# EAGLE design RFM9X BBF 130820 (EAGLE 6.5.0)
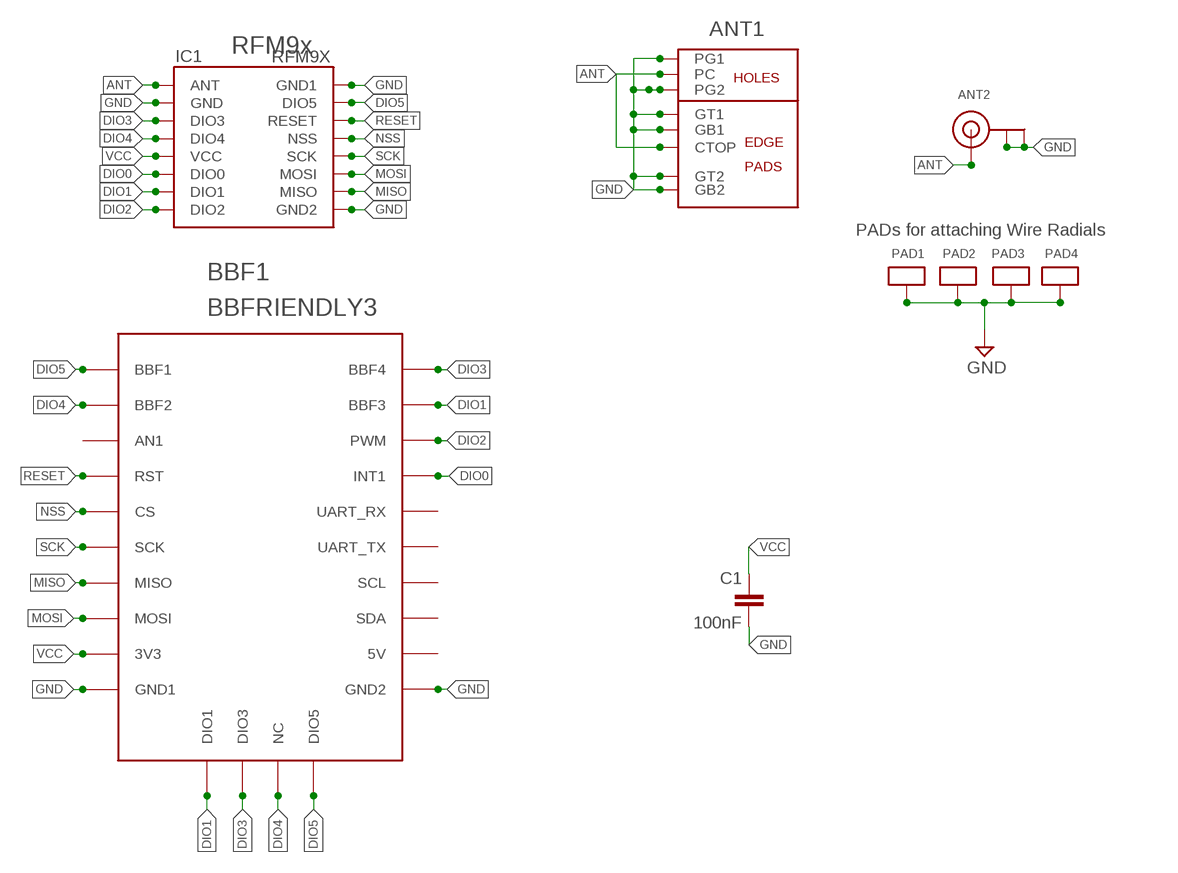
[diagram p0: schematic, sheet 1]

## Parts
ANT1  CUSTOMSMA  [CUSTOMSMA]
ANT2  ANTENNA_U.FL  [U.FL]
BBF1  BBFRIENDLY3  [PCB_SOCKET_BBFRIENDLY3]
C1  100nF  C-EUC1206  [C1206]
IC1  RFM9X  RFM98_PIH  [RFM98_PIH]
PAD1  ANTPAD2  [ANTPAD2]
PAD2  ANTPAD2  [ANTPAD2]
PAD3  ANTPAD2  [ANTPAD2]
PAD4  ANTPAD2  [ANTPAD2]

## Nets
ANT: ANT1.CTOP ANT1.PC ANT2.3(SIGNAL) IC1.ANT
DIO0: BBF1.INT(INT1) IC1.DIO0
DIO1: BBF1.BBF3 BBF1.DIO1 IC1.DIO1
DIO2: BBF1.PWM IC1.DIO2
DIO3: BBF1.BBF4 BBF1.DIO3 IC1.DIO3
DIO4: BBF1.BBF2 BBF1.NC IC1.DIO4
DIO5: BBF1.BBF1 BBF1.DIO5 IC1.DIO5
GND [VDD]: ANT1.G1 ANT1.G2 ANT1.GB1 ANT1.GB2 ANT1.GT1 ANT1.GT2 ANT2.1(GND) ANT2.2(GND) BBF1.GND1 BBF1.GND2 C1.2 IC1.GND IC1.GND1 IC1.GND2 PAD1.P$1 PAD2.P$1 PAD3.P$1 PAD4.P$1
MISO: BBF1.MISO IC1.MISO
MOSI: BBF1.MOSI IC1.MOSI
NSS: BBF1.CS IC1.NSS
RESET: BBF1.RST IC1.RESET
SCK: BBF1.SCK IC1.SCK
VCC [VDD]: BBF1.3V3 C1.1 IC1.VCC
Unconnected: BBF1.5V BBF1.AN1 BBF1.RX(UART_RX) BBF1.SCL BBF1.SDA BBF1.TX(UART_TX)

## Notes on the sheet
- RFM9x
- PADs for attaching Wire Radials

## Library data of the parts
ANT1 = con-coax:CUSTOMSMA
ANT2 = adafruit:ANTENNA_U.FL: U.FL Antenna Connector
BBF1 = My_Mikrobus:BBFRIENDLY3
C1 = resistor:C-EU: CAPACITOR, European symbol
IC1 = LMA2:RFM98_PIH
PAD1-PAD4 = LMA2:ANTPAD2

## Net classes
0 default: width 0.152 mm
1 POWER: width 0.508 mm
2 VDD: width 0.508 mm

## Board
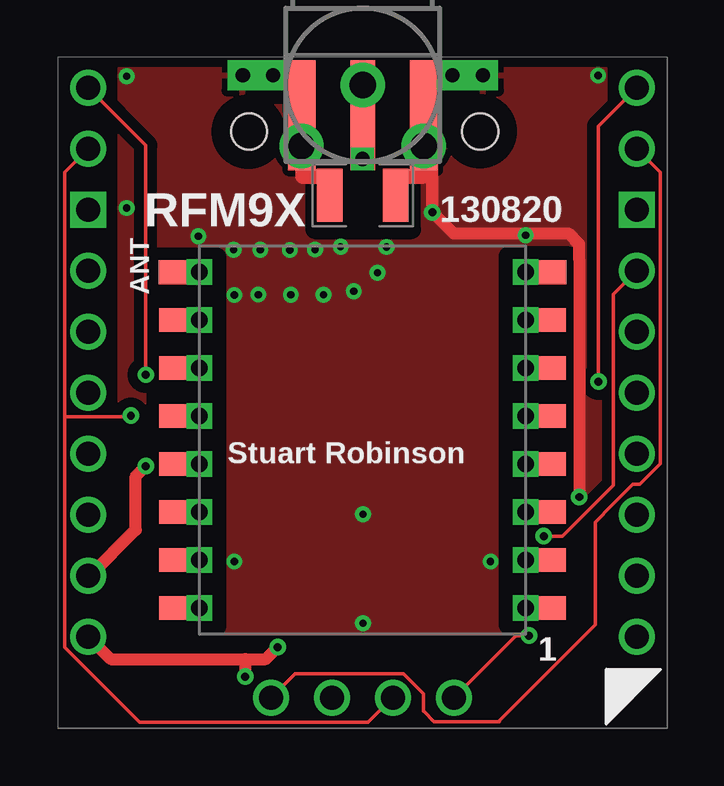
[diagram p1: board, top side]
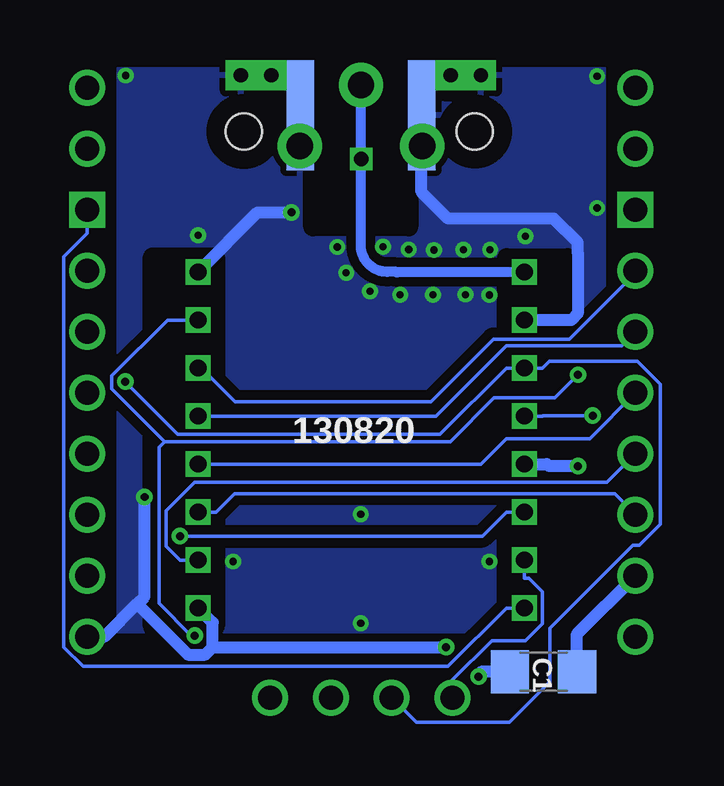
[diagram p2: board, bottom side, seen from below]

No outline drawn. Coordinates in mm, seen from the top.
Copper layers (1*16): Top 0.0356mm / dielectric 1.5011mm / Bottom 0.0356mm
Design rules "LaenPCBOrder *": minimum track width 6mil, minimum drill 13mil, track to track 6mil, track to pad 6mil, pad to pad 6mil, via to via 6mil, smd to smd 6mil, copper to edge 15mil, drill to drill 6mil, minimum pad ring 7mil, minimum via ring 7mil, stop-mask expansion 4mil, vias tented up to drill 1000mil, thermal gap 10mil
Holes 1.5 mm at 7.97,24.85 17.6,24.85
tRestrict: area 16.5,23.8 to 18.7,26; area 6.8,23.8 to 9,25.9; area 10.7,20.8 to 14.8,24; area 4.1,4.2 to 6.6,19.6; area 18.8,4.3 to 21.3,19.7; area 10.7,23.1 to 14.8,27.8; area 8.5,26.4 to 9.2,26.5; area 16.2,26.4 to 16.6,26.6; area 15.8,25.4 to 15.9,25.7
bRestrict: area 10.7,20.9 to 14.7,28; area 6.9,23.8 to 9,25.9; area 16.5,23.7 to 18.7,26; area 4.1,4.2 to 6.6,19.6; area 18.8,4.2 to 21.4,19.6; area 16.2,26.5 to 16.7,26.6; area 15.8,25.3 to 15.9,25.8; area 8.6,26.5 to 9.2,26.6

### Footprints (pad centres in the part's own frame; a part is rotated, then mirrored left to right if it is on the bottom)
CUSTOMSMA = smd 4.572 x 1.016: CTOP -1.27,0 | drill 1.1 pad 1.85: G1 -2.55,2.55; G2 -2.55,-2.55; PC 0,0 | smd 4.572 x 1.143 bottom: GB1 -1.27,2.54; GB2 -1.27,-2.54 | smd 4.572 x 1.143: GT1 -1.27,2.54; GT2 -1.27,-2.54
U.FL = smd 2.2 x 1.05: 1 0,1.375; 2 0,-1.375 | smd 0.8 x 1: 3 1.525,0
PCB_SOCKET_BBFRIENDLY3 = drill 1: 3V3 -11.43,3.81; 5V 11.43,3.81; BBF1 -11.43,24.13; BBF2 -11.43,21.59; BBF3 11.43,21.59; BBF4 11.43,24.13; CS -11.43,13.97; DIO1 -3.81,-1.27; DIO3 -1.27,-1.27; DIO5 3.81,-1.27; GND1 -11.43,1.27; GND2 11.43,1.27; INT 11.43,16.51; MISO -11.43,8.89; MOSI -11.43,6.35; NC 1.27,-1.27; RST -11.43,16.51; RX 11.43,13.97; SCK -11.43,11.43; SCL 11.43,8.89; SDA 11.43,6.35; TX 11.43,11.43 | drill 1 square: AN1 -11.43,19.05; PWM 11.43,19.05
C1206 = smd 1.6 x 1.8: 1 -1.4,0; 2 1.4,0
RFM98_PIH = drill 0.7 pad 0.965 square: ANT -6.8,7.5; DIO0 -6.8,-2.5; DIO1 -6.8,-4.5; DIO2 -6.8,-6.5; DIO3 -6.8,3.5; DIO4 -6.8,1.5; DIO5 6.8,5.5; GND -6.8,5.5; GND2 6.8,-6.5; MISO 6.8,-4.5; MOSI 6.8,-2.5; NSS 6.8,1.5; RESET 6.8,3.5; SCK 6.8,-0.5; VCC -6.8,-0.5 | drill 0.7 pad 1.016 square: GND1 6.8,7.5 | smd 2.2 x 1: P$2 -7.4,7.5; P$6 7.4,7.5 | smd 2.159 x 0.965: P$4 -7.4,5.5; P$5 -7.4,1.5; P$7 7.4,5.5; P$9 -7.4,3.5; P$10 -7.4,-0.5; P$11 -7.4,-2.5; P$12 -7.4,-4.5; P$13 -7.4,-6.5; P$14 7.4,-6.5; P$15 7.4,-4.5; P$16 7.4,-2.5; P$17 7.4,-0.5; P$18 7.4,1.5; P$19 7.4,3.5
ANTPAD2 = drill 0.6 pad 1.27 square: P$1 0,0

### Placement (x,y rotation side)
ANT1  12.71,26.8 90 top
ANT2  12.71,22.2 90 top
BBF1  12.7,2.54 0 top
C1  5.1,2.34 180 bottom
IC1  12.7,11.5 0 top
PAD1  8.97,27.2 0 top
PAD2  7.71,27.2 0 top
PAD3  16.45,27.2 0 top
PAD4  17.72,27.2 0 top

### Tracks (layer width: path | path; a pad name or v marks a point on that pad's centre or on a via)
ANT
  Top 0.152: ANT2.3 12.71,24.35 ANT1.CTOP ANT1.PC
  Bottom 0.406: IC1.ANT 11.21,18.99 arc90 11.23,19.01 11.62,19.01 arc90 12.72,20.11 ANT1.PC arc90 ANT1.PC
DIO0  (via drill 0.33 pad 0.69)
  Top 0.152: BBF1.INT 23.15,18.07 23.15,10.12 21.04,8 v20.26,8
  Bottom 0.152: IC1.DIO0 6.66,9 7.66,8 v20.26,8
DIO1
  Top 0.152: BBF1.DIO1 9.88,2.26 14.4,2.26 15.24,1.42 15.24,1.14 15.25,1.14 15.25,0.69 15.26,0.69 15.69,0.26 18.4,0.26 18.4,0.3 22.4,4.3 22.4,8.58 23.12,9.3 23.98,10.16 24.26,10.16 25.11,11.01 25.11,23.15 BBF1.BBF3
  Bottom 0.152: BBF1.DIO1 8.89,2 7.25,3.64 5.85,3.64 5.14,4.35 5.14,5.68 5.71,6.24 5.9,6.24 IC1.DIO1
DIO2
  Bottom 0.152: IC1.DIO2 6.66,5 9.09,2.57 24.3,2.57 25.11,3.38 25.11,19.63 24.13,20.61 BBF1.PWM
DIO3  (via drill 0.33 pad 0.69)
  Top 0.152: BBF1.BBF4 22.54,25.08 v22.54,14.43
  Bottom 0.152: BBF1.DIO3 10.4,0.24 6.53,0.24 4.84,1.93 4.84,4.17 1.38,7.62 1.11,7.62 0.24,8.49 0.24,14.33 1.2,15.29 4.85,15.29 5.14,15 IC1.DIO3 6.66,15 9.41,12.24 20.35,12.24 v22.54,14.43
DIO4  (via drill 0.33 pad 0.69)
  Top 0.152: 0.29,12.97 0.29,23.15 BBF1.BBF2 | BBF1.NC 12.94,0.24 3.42,0.24 0.29,3.37 0.29,12.97 | 0.29,12.97 2.99,12.97 v3.04,13.02
  Bottom 0.152: IC1.DIO4 5.14,13 5.12,13.02 v3.04,13.02
DIO5  (via drill 0.33 pad 0.69)
  Top 0.152: v3.66,14.72 3.66,24.28 BBF1.BBF1 | BBF1.DIO5 19.09,3.85 v19.64,3.85
  Bottom 0.152: 20.9,11.94 8.99,11.94 7.17,13.76 4.62,13.76 v3.66,14.72 | IC1.DIO5 20.78,17 23.11,14.67 23.11,14.14 20.9,11.94 | 20.9,11.94 21.14,11.71 21.14,5.19 19.8,3.85 v19.64,3.85
GND  (via drill 0.3, 0.33 pad 0.69)
  Top 0.508: ANT1.GB2 ANT1.G2 15.62,23.89 v15.62,21.48 16.49,20.61 | 7.81,2.87 8.66,2.87 v9.16,3.37 | BBF1.GND1 2.21,2.87 7.81,2.87 | 7.81,2.87 v7.81,2.14 | 16.49,20.61 | 16.49,20.61 20.67,20.61 21.11,20.61 21.28,20.61 21.73,20.16 21.73,19.55 21.74,19.54 v21.74,9.63 | 10.2,24.21 10.2,24.1 | 11.3,23 ANT2.1 | PAD2.P$1 8.75,27.2 | ANT1.G1 10.2,24.21 | 10.2,24.21 ANT1.GB1 | 14.1,23 ANT2.2
  Top 0.635: PAD1.P$1 10.17,27.2 ANT1.GB1 | PAD3.P$1 15.25,27.2 ANT1.GB2 | 10.2,24.1 10.21,24.1 10.21,22.99 11.3,22.99 11.3,23 | 14.1,23 15.26,23 ANT1.G2
  Bottom 0.508: C1.2 7.71,2.34 7.71,2.25 v7.81,2.14 | 22.04,5.18 21.74,5.48 v21.74,9.63 | 18.89,3.37 v9.16,3.37 | 22.04,5.18 19.92,3.06 19.2,3.06 18.89,3.37 | 18.89,3.37 18.89,4.39 IC1.GND2 | IC1.GND 3.95,17 3.67,17.27 3.67,19.82 3.67,20.22 4.68,21.23 9.08,21.23 10.18,22.33 10.18,24.23 ANT1.G1 10.29,24.38 10.29,25.41 ANT1.GB1 | BBF1.GND2 23.41,3.81 22.04,5.18 | ANT1.G2 15.26,25.4 15.25,25.41 ANT1.GB2 | IC1.GND1 17.02,21.48 v15.62,21.48
  other vias: 7.33,19.93 7.36,18.04 8.44,19.93 8.36,18.06 9.67,19.92 9.71,18.05 10.72,19.94 12.34,18.2 11.08,18.05 13.33,18.97 13.7,20.04 11.79,20.05 2.87,27.16 22.52,27.19 19.5,20.53 5.86,20.49 7.36,6.94 18.04,6.94 12.72,8.91 12.72,4.37 2.87,21.67
  pour Bottom (isolate 0.4): 2.54,27.5 22.86,27.5 22.86,4 2.54,4
  pour Top (isolate 0.4): 2.54,27.5 22.86,27.5 22.86,4 2.54,4
MISO
  Bottom 0.152: IC1.MISO 20.26,7 20.83,7.58 20.83,9.06 19.65,10.24 2.46,10.24 BBF1.MISO
MOSI
  Bottom 0.152: IC1.MOSI 18.74,9 17.99,9.76 2.14,9.76 BBF1.MOSI
N$1  (via drill 0.6 pad 0.69)
  other vias: 12.7,23.71
NSS
  Bottom 0.152: BBF1.CS 1.84,15.94 6.66,15.94 9.6,13 IC1.NSS
RESET
  Bottom 0.152: BBF1.RST 1.27,18.95 3.98,16.24 4.03,16.2 7.19,16.2 9.79,13.6 10.08,13.6 17.96,13.6 19.36,15 IC1.RESET
SCK
  Bottom 0.152: BBF1.SCK 3.18,12.06 6.65,12.06 7.71,11 18.74,11 IC1.SCK
VCC  (via drill 0.33 pad 0.69)
  Top 0.508: BBF1.3V3 1.34,6.35 3.25,8.26 3.25,10.5 v3.66,10.91
  Bottom 0.508: C1.1 3.7,3.92 BBF1.3V3 | IC1.VCC 4.97,11 4.88,10.91 v3.66,10.91

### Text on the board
tPlace: RFM9X | 130820 | ANT | Stuart Robinson | 1
bPlace: 130820 | C1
